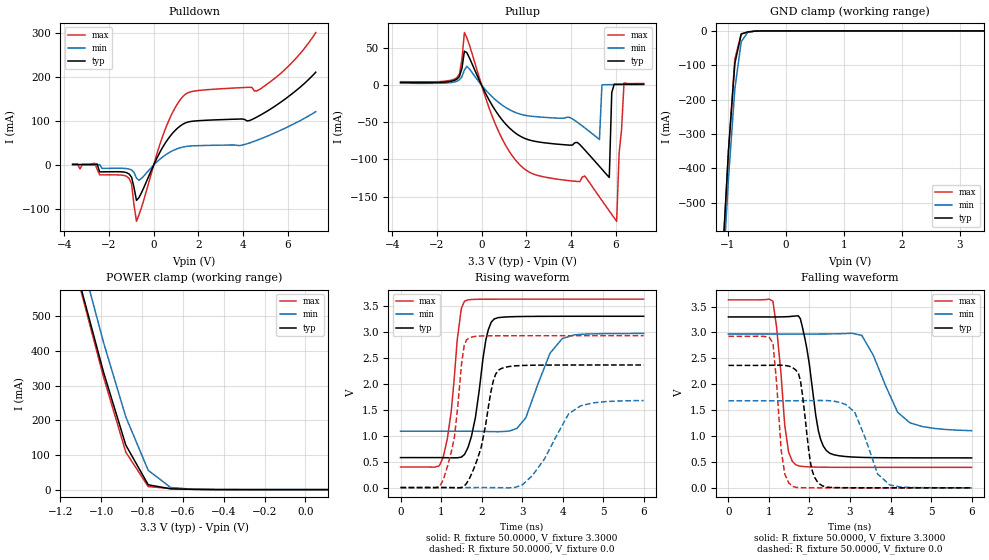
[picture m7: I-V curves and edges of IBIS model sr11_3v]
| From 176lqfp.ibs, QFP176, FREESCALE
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[Model] sr11_3v
|   Model sr11_3v
Model_type 3-state
Polarity   Non-Inverting
Enable   Active-High
Vmeas = 1.65
C_comp   4.7070pF   4.5257pF   4.9713pF
[Temperature Range]   25.0000   0.1500k   -40.0000
[Voltage Range]   3.3000V   2.9700V   3.6300V
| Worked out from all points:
|   slope of the pulldown table from 0 to 0.495 V, typ, clamps not added: 10.3 ohm
|   slope of the pullup table from 0 to 0.495 V, typ, clamps not added: 17.6 ohm
|   GND clamp passes 1 mA (typ) near -0.56 V on its own axis
|   POWER clamp passes 1 mA (typ) near -0.57 V on its own axis
|   rising waveform, R_fixture 50.0000, V_fixture 3.3000: 20-80 % time 301ps typ, 548ps min, 248ps max; typ from 0.577 V to 3.3 V
|   rising waveform, R_fixture 50.0000, V_fixture 0.0: 20-80 % time 382ps typ, 741ps min, 282ps max; typ from 0 V to 2.36 V
|   falling waveform, R_fixture 50.0000, V_fixture 3.3000: 20-80 % time 296ps typ, 618ps min, 218ps max; typ from 3.3 V to 0.578 V
|   falling waveform, R_fixture 50.0000, V_fixture 0.0: 20-80 % time 219ps typ, 474ps min, 177ps max; typ from 2.36 V to 0 V
[Pulldown]
|Voltage   I(typ)   I(min)   I(max)
-3.63V    1.36mA     780uA      2.26mA
-3.3V     1.318mA    753uA      -8.762mA
-2.64V    1.346mA    691uA      4.191mA
-2.42V    -15.32mA   1.261mA    -22.16mA
-1.1V     -20.24mA   -9.013mA   -30.21mA
-990mV    -27.45mA   -11.16mA   -42.69mA
-770mV    -80.32mA   -29.55mA   -127.8mA
440mV     43.55mA    19.89mA    70.89mA
1.32V     93.29mA    41.11mA    156.5mA
4.62V     109.2mA    56.28mA    168.7mA
6.05V     156.3mA    87.92mA    225.7mA
7.26V     211.2mA    121.5mA    301.3mA
[Pullup]
|Voltage   I(typ)   I(min)   I(max)
-3.63V    3.6mA      2.54mA     4.7mA
-1.1V     8.214mA    5.392mA    10.32mA
-770mV    45.78mA    20.45mA    70.83mA
1.54V     -64.99mA   -37.01mA   -101.5mA
5.28V     -109.4mA   -73.1mA    -150.6mA
5.39V     -113.1mA   334uA      -155.3mA
5.72V     -124.2mA   703uA      -169.3mA
5.83V     -10.04mA   715uA      -174mA
6.05V     1.218mA    735uA      -183.3mA
6.16V     1.244mA    744uA      -91.77mA
6.38V     1.286mA    761uA      3.046mA
7.26V     1.41mA     830uA      2.26mA
[GND_clamp]
|Voltage   I(typ)   I(min)   I(max)
-3.63V    -10.38A    -10.28A    -10.54A
-1.1V     -683.5mA   -753.4mA   -695.2mA
-990mV    -349.5mA   -429.8mA   -348.6mA
-880mV    -94.6mA    -168.5mA   -81.77mA
-770mV    -9.279mA   -31.37mA   -8.241mA
-660mV    -2.916mA   -4.583mA   -4.405mA
-440mV    -65.66uA   -239.8uA   -36.5uA
3.41V     626.5pA    220.2uA    6.002pA
[POWER_clamp]
|Voltage   I(typ)   I(min)   I(max)
-3.63V    7.308A     7.439A     7.307A
-1.1V     583.2mA    670.8mA    574.6mA
-990mV    341mA      426.7mA    326.9mA
-880mV    128.5mA    209.9mA    108.2mA
-770mV    13.88mA    55.46mA    8.675mA
-660mV    2.265mA    6.121mA    3.037mA
-550mV    681.9uA    981.3uA    900.8uA
110mV     37.89pA    5.502nA    6.134pA
[Ramp]
| variable   typ   min   max
dV/dt_r  1.4171/0.3817n   1.0060/0.7104n   1.7552/0.2808n
dV/dt_f  1.6329/0.2964n   1.1196/0.6043n   1.9404/0.2050n
R_load = 50.0000
[Rising Waveform]
R_fixture= 50.0000
V_fixture= 3.3000
V_fixture_min= 2.9700
V_fixture_max= 3.6300
|time   V(typ)   V(min)   V(max)
0s        577.1mV    1.085V     395.9mV
1.053ns   576.5mV    1.085V     581.8mV
1.501ns   586mV      1.085V     3.456V
1.578ns   637.1mV    1.085V     3.589V
1.849ns   1.353V     1.084V     3.626V
2.105ns   2.843V     1.081V     3.629V
2.31ns    3.247V     1.077V     3.629V
3.091ns   3.296V     1.343V     3.63V
3.99ns    3.299V     2.869V     3.63V
6ns       3.3V       2.969V     3.63V
[Rising Waveform]
R_fixture= 50.0000
V_fixture= 0.0
V_fixture_min= 0.0
V_fixture_max= 0.0
|time   V(typ)   V(min)   V(max)
0s        4.319nV    133.6nV    3.708nV
1.059ns   712.6uV    42.97uV    154.3mV
1.33ns    -2.563mV   19.88uV    975.3mV
1.572ns   28.72mV    75.83uV    2.742V
1.712ns   191.8mV    185.3uV    2.888V
1.989ns   771.2mV    514.5uV    2.92V
2.432ns   2.27V      -1.889mV   2.925V
3.248ns   2.357V     226.4mV    2.925V
4.447ns   2.361V     1.576V     2.925V
6ns       2.362V     1.677V     2.925V
[Falling Waveform]
R_fixture= 50.0000
V_fixture= 3.3000
V_fixture_min= 2.9700
V_fixture_max= 3.6300
|time   V(typ)   V(min)   V(max)
0s        3.3V       2.97V      3.63V
1.097ns   3.3V       2.97V      3.604V
1.388ns   3.303V     2.97V      1.217V
1.658ns   3.318V     2.97V      446.4mV
1.819ns   3.125V     2.97V      414.7mV
2.219ns   1.102V     2.97V      399.9mV
2.415ns   721.1mV    2.971V     397.8mV
3.292ns   588mV      2.943V     396.1mV
4.475ns   579.9mV    1.257V     396mV
6ns       578.5mV    1.104V     395.9mV
[Falling Waveform]
R_fixture= 50.0000
V_fixture= 0.0
V_fixture_min= 0.0
V_fixture_max= 0.0
|time   V(typ)   V(min)   V(max)
0s        2.364V     1.681V     2.925V
1.099ns   2.367V     1.68V      2.794V
1.3ns     2.368V     1.681V     733.8mV
1.579ns   2.325V     1.681V     29.07mV
1.777ns   2.066V     1.683V     3.925mV
2.075ns   310.8mV    1.685V     1.128mV
2.321ns   37.2mV     1.686V     467.2uV
3.115ns   1.624mV    1.465V     104uV
3.98ns    620uV      55.77mV    7.183uV
6ns       199.8uV    915.6uV    6.657uV
